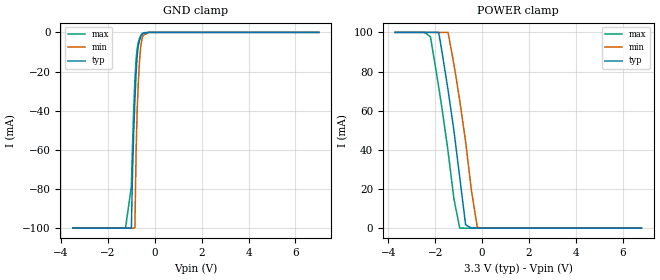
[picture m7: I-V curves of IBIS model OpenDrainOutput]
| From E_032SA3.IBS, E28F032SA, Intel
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|********************Open Drain Output Model************************
[Model]   OpenDrainOutput
Model_type   Open_drain
|   for RY/BY# pin 53
Vinl = 0.8V
Vinh = 2.0V
| Variable   typ   min   max
C_comp   9.61p   NA   11.6p
[Voltage Range]   3.3V   3.0V   3.6V
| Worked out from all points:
|   GND clamp passes 1 mA (typ) near -0.54 V on its own axis
|   POWER clamp passes 1 mA (typ) near -0.59 V on its own axis
[Pulldown]
| [Pullup] and [Pulldown] IV curves include only the current through
| the channels of output driver transistors when outputs are enabled
| with OE# = VIL.  Although the output driver transistors have np and
| pn diodes inherently created by CMOS IC fabrication between the
| drain and bulk of n-channel and p-channel CMOS transistors,
| the current through these junction diodes is not included in
| [Pullup] or [Pulldown].  Instead that drain/bulk diode current is
| included in the [POWER_clamp] or [GND_clamp] sections, which are
| not dependent on the state of OE# or output data value.  The RY/BY#
| Pulldown information is not provided for this device.  The table
| below is for the compatibility with some IBIS parsers.
|Voltage  I(typ)   I(min)   I(max)
-5V       0A         0A         0A
10V       0A         0A         0A
[GND_clamp]
| [POWER_clamp] and [GND_clamp] IV curves describe ESD protection
| circuits PLUS some np and pn diodes which exist between the
| drain and bulk of n-channel and p-channel CMOS transistors.
| These drain/bulk diodes are inherent in CMOS IC fabrication,
| and are visible on the node of the I/O pin at all times.
| Even the drain/bulk diodes of output driver [Pullup] and [Powerdown]
| transistors are included in [POWER_clamp] or [GND_clamp], because
| these diodes contribute to I/O pin current even when the
| chip outputs are tristated by OE# = VIH.
| For example, when V forced on the I/O pin is large, we are
| forward biasing the pn diode at the drain/bulk interface in the
| p-channel pullup transistor.  Similarly, when V forced on the
| I/O pin is sufficiently negative with respect to the substrate
| ground, we are forward biasing the np diode at the drain/bulk
| interface in the n-channel pulldown transistor.  The effects
| of these diodes are included in [POWER_clamp] or [GND_clamp].
|Voltage  I(typ)   I(min)   I(max)
-3.5V     -99.84mA   -99.84mA   -99.85mA
-1.25V    -99.84mA   -99.84mA   -99.85mA
-1V       -99.84mA   -99.84mA   -78.52mA
-950mV    -71.19mA   -99.84mA   -57.54mA
-900mV    -50.96mA   -99.84mA   -39.26mA
-850mV    -34.78mA   -99.62mA   -24.43mA
-800mV    -21.1mA    -61.65mA   -13.82mA
-750mV    -11.75mA   -38.54mA   -8.01mA
-650mV    -3.891mA   -14.15mA   -2.999mA
-600mV    -2.235mA   -7.162mA   -1.606mA
-500mV    -459.6uA   -1.565mA   -211.6uA
7V        0A         0A         0A
[Pullup]
| (Voltages for [Pullup] and [POWER_clamp] are specified with
| negative respect to Vcc.  Reference the IBIS documentation
| for more information regarding Vtable = Vcc - Voutput.
| This method keeps -Vds constant for the values in all three
| columns across a line of the table.)
| [Pullup] and [Pulldown] IV curves include only the current through
| the channels of output driver transistors when outputs are enabled
| with OE# = VIL.  Although the output driver transistors have np and
| pn diodes inherently created by CMOS IC fabrication between the
| drain and bulk of n-channel and p-channel CMOS transistors,
| the current through these junction diodes is not included in
| [Pullup] or [Pulldown].  Instead that drain/bulk diode current is
| included in the [POWER_clamp] or [GND_clamp] sections, which are
| not dependent on the state of OE# or output data value.
|   Voltage  I(typ)   I(min)   I(max)
-5V       0A         0A         0A
10V       0A         0A         0A
[POWER_clamp]
| (Voltages for [Pullup] and [POWER_clamp] are specified with
| negative respect to Vcc.  Reference the IBIS documentation
| for more information regarding Vtable = Vcc - Voutput.
| This method keeps -Vds constant for the values in all three
| columns across a line of the table.
| [POWER_clamp] and [GND_clamp] IV curves describe ESD protection
| circuits PLUS some np and pn diodes which exist between the
| drain and bulk of n-channel and p-channel CMOS transistors.
| These drain/bulk diodes are inherent in CMOS IC fabrication,
| and are visible on the node of the I/O pin at all times.
| Even the drain/bulk diodes of output driver [Pullup] and [Powerdown]
| transistors are included in [POWER_clamp] or [GND_clamp], because
| these diodes contribute to I/O pin current even when the
| chip outputs are tristated by OE# = VIH.
| For example, when V forced on the I/O pin is large, we are
| forward biasing the pn diode at the drain/bulk interface in the
| p-channel pullup transistor.  Similarly, when V forced on the
| I/O pin is sufficiently negative with respect to the substrate
| ground, we are forward biasing the np diode at the drain/bulk
| interface in the n-channel pulldown transistor.  The effects
| of these diodes are included in [POWER_clamp] or [GND_clamp].
|Voltage  I(typ)   I(min)   I(max)
-3.7V     100mA      100mA      100mA
-2.45V    100mA      100mA      100mA
-2.2V     100mA      100mA      97.77mA
-1.85V    100mA      100mA      72.28mA
-1.7V     89.53mA    100mA      60.56mA
-1.45V    70.71mA    100mA      39.43mA
-1.2V     50.02mA    83.94mA    15.16mA
-950mV    26mA       65.25mA    36.7uA
-700mV    1.736mA    44.18mA    0A
-450mV    0A         19.11mA    0A
-200mV    0A         387.4uA    0A
6.8V      0A         0A         0A
[Ramp]
| The RY/BY# Ramp information is not provided for this devide.  The table
| below is for the compatibility with some IBIS parsers.
|Variable   typ   min   max
dV/dt_r   0V/0ns   0V/0ns   0V/0ns
dV/dt_f   0V/0ns   0V/0ns   0V/0ns
